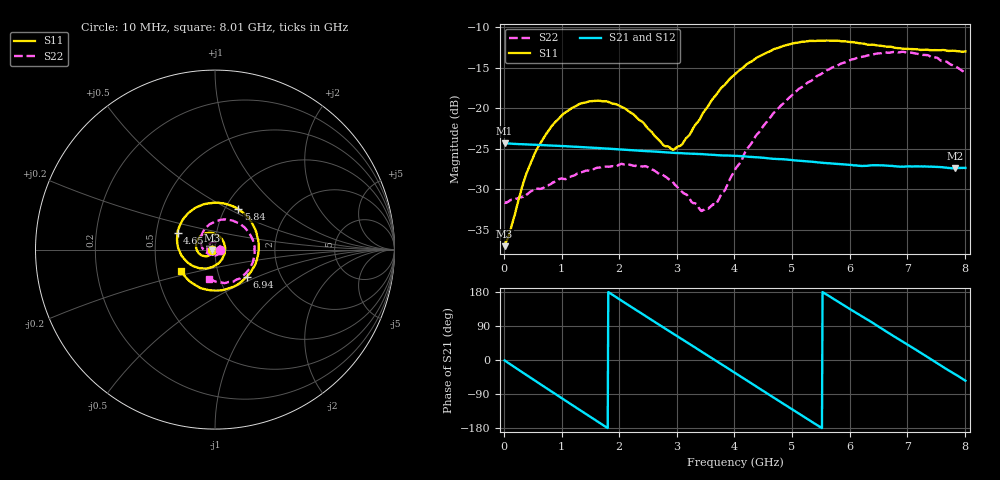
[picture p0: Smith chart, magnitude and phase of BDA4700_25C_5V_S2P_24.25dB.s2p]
!Agilent Technologies,E5071B,MY42404982,A.09.10
!Date: Mon Oct 20 13:38:39 2025
!Data & Calibration Information:
!Freq	S11:SOLT2(ON)	S21:SOLT2(ON)	S12:SOLT2(ON)	S22:SOLT2(ON)
# Hz S RI R 50
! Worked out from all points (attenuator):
!   801 points, 10 MHz to 8.01 GHz, reference 50 ohm
!   highest |S21| = -24.33 dB at 10 MHz (marker M1); lowest = -27.4 dB at 7.83 GHz (marker M2)
!   lowest |S11| = -37.0 dB at 10 MHz (marker M3), VSWR 1.03, Z = 48.6 - j0.137 ohm
!   |S11| at or under -10 dB: start of sweep to end of sweep
!   |S22| runs from -32.7 to -13.0 dB; largest |S21 - S12| = 0.00051
!   S11 on the Smith chart (normalised r, x): 10 MHz: 0.97, -0.00; 4.65 GHz: 0.65, +0.13; 5.84 GHz: 1.16, +0.56; 6.94 GHz: 1.35, -0.43; 8.01 GHz: 0.66, -0.17
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1e7  -0.014 -0.00141  0.0608 -0.00128  0.0608 -0.00134  0.0261 -0.000855
1e8  -0.0152 -0.00807  0.0594 -0.011  0.0594 -0.011  0.0266 -0.0048
3.6e8  -0.0255 -0.0267  0.048 -0.0357  0.048 -0.0358  0.022 -0.0184
5.8e8  -0.0433 -0.0366  0.0309 -0.0507  0.0309 -0.0507  0.014 -0.0286
9.9e8  -0.0859 -0.0242  -0.00971 -0.0576  -0.00972 -0.0577  -0.0141 -0.0339
1.35e9  -0.1062 0.0169  -0.0409 -0.0405  -0.0409 -0.0405  -0.0362 -0.0178
1.98e9  -0.0533 0.0899  -0.0532 0.0167  -0.0533 0.0168  -0.0339 0.0286
2.68e9  0.0482 0.0424  -0.00412 0.0537  -0.00411 0.0536  0.013 0.0374
2.97e9  0.0547 -0.0133  0.0212 0.0485  0.0212 0.0485  0.0258 0.0214
3.44e9  -0.00392 -0.0914  0.0486 0.0187  0.0486 0.0186  0.0184 -0.0143
3.69e9  -0.0617 -0.1052  0.0513 -0.00275  0.0513 -0.00288  0.000334 -0.0258
4.01e9  -0.141 -0.08  0.0422 -0.0284  0.0422 -0.0285  -0.0325 -0.0258
4.65e9  -0.2084 0.0927  -0.00533 -0.0485  -0.00522 -0.0486  -0.0792 0.0435
4.97e9  -0.1619 0.1886  -0.029 -0.0383  -0.0289 -0.0384  -0.0682 0.0961
5.35e9  -0.047 0.256  -0.0448 -0.0132  -0.0448 -0.0134  -0.0153 0.1482
5.84e9  0.1305 0.2242  -0.0392 0.0226  -0.0391 0.0226  0.0938 0.1626
6.25e9  0.2284 0.1022  -0.0167 0.0407  -0.0162 0.0409  0.18 0.106
6.68e9  0.2307 -0.0655  0.0143 0.0417  0.0144 0.0418  0.2205 -0.000138
6.94e9  0.1763 -0.152  0.0297 0.0319  0.0299 0.0318  0.211 -0.0713
7.37e9  0.0252 -0.2279  0.0434 0.0046  0.0434 0.00452  0.1364 -0.162
7.83e9  -0.1449 -0.1735  0.0339 -0.0257  0.0339 -0.0259  0.0125 -0.1815
8.01e9  -0.1895 -0.1198  0.0248 -0.0349  0.0249 -0.0348  -0.0309 -0.1619
